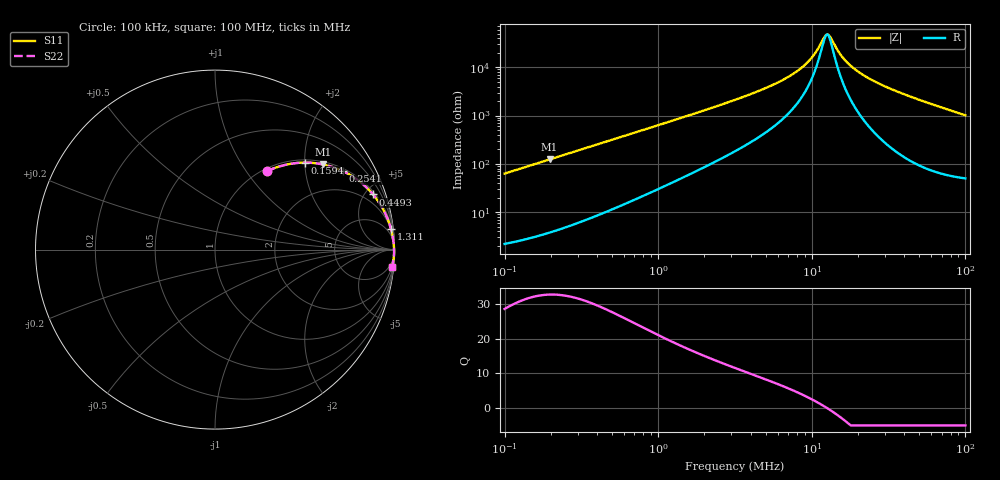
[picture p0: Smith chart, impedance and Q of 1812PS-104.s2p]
# MHz S MA R 50
!Freq  MagS11  AngS11  MagS21  AngS21  MagS12  AngS12  MagS22  AngS22
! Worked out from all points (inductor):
!   801 points, 100 kHz to 100 MHz, reference 50 ohm
!   read as one part in series: L = 100 uH near 103.5 kHz
!   highest Q = 32.7 at 196.1 kHz (marker M1), where L = 100 uH
!   self-resonance near 12.48 MHz
!   S11 on the Smith chart (normalised r, x): 100 kHz: 1.04, +1.26; 159.4 kHz: 1.06, +2.00; 254.1 kHz: 1.10, +3.19; 449.3 kHz: 1.20, +5.65; 1.311 MHz: 2, +17; 100 MHz: 2, -20
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0.1  0.524 56.4  0.8336 -31.6  0.8336 -31.6  0.524 56.4
0.1594043  0.697 44.1  0.6957 -44.2  0.6957 -44.2  0.697 44.1
0.1961101  0.7652 38.4  0.6208 -49.9  0.6208 -49.9  0.7652 38.4
0.2540973  0.836 31.5  0.5235 -56.7  0.5235 -56.7  0.836 31.5
0.3180534  0.8831 26.2  0.4417 -62.0  0.4417 -62.0  0.8831 26.2
0.4492623  0.9325 19.3  0.33 -68.7  0.33 -68.7  0.9325 19.3
1.002882  0.9806 8.9  0.1548 -78.4  0.1548 -78.4  0.9806 8.9
1.31069  0.9866 6.8  0.1187 -80.1  0.1187 -80.1  0.9866 6.8
3.162278  0.9948 2.7  0.04708 -82.4  0.04708 -82.4  0.9948 2.7
4.911905  0.9964 1.6  0.02755 -81.7  0.02755 -81.7  0.9964 1.6
6.702703  0.9971 1.0  0.01718 -79.7  0.01718 -79.7  0.9971 1.0
8.462526  0.9975 0.6  0.01057 -75.7  0.01057 -75.7  0.9975 0.6
10.05773  0.9977 0.3  0.006148 -67.7  0.006148 -67.7  0.9977 0.3
12.16186  0.9979 0.0  0.002286 -22.0  0.002286 -22.0  0.9979 0.0
12.80855  0.9979 -0.0  0.00212 12.2  0.00212 12.2  0.9979 -0.0
13.25867  0.998 -0.1  0.002433 32.8  0.002433 32.8  0.998 -0.1
15.48817  0.9981 -0.3  0.005622 69.7  0.005622 69.7  0.9981 -0.3
18.09256  0.9981 -0.5  0.009548 78.5  0.009548 78.5  0.9981 -0.5
22.84283  0.9982 -0.9  0.01606 82.9  0.01606 82.9  0.9982 -0.9
31.71393  0.998 -1.5  0.02686 84.9  0.02686 84.9  0.998 -1.5
51.88  0.9967 -2.8  0.04895 84.7  0.04895 84.7  0.9967 -2.8
100  0.9904 -5.6  0.09793 81.6  0.09793 81.6  0.9904 -5.6
